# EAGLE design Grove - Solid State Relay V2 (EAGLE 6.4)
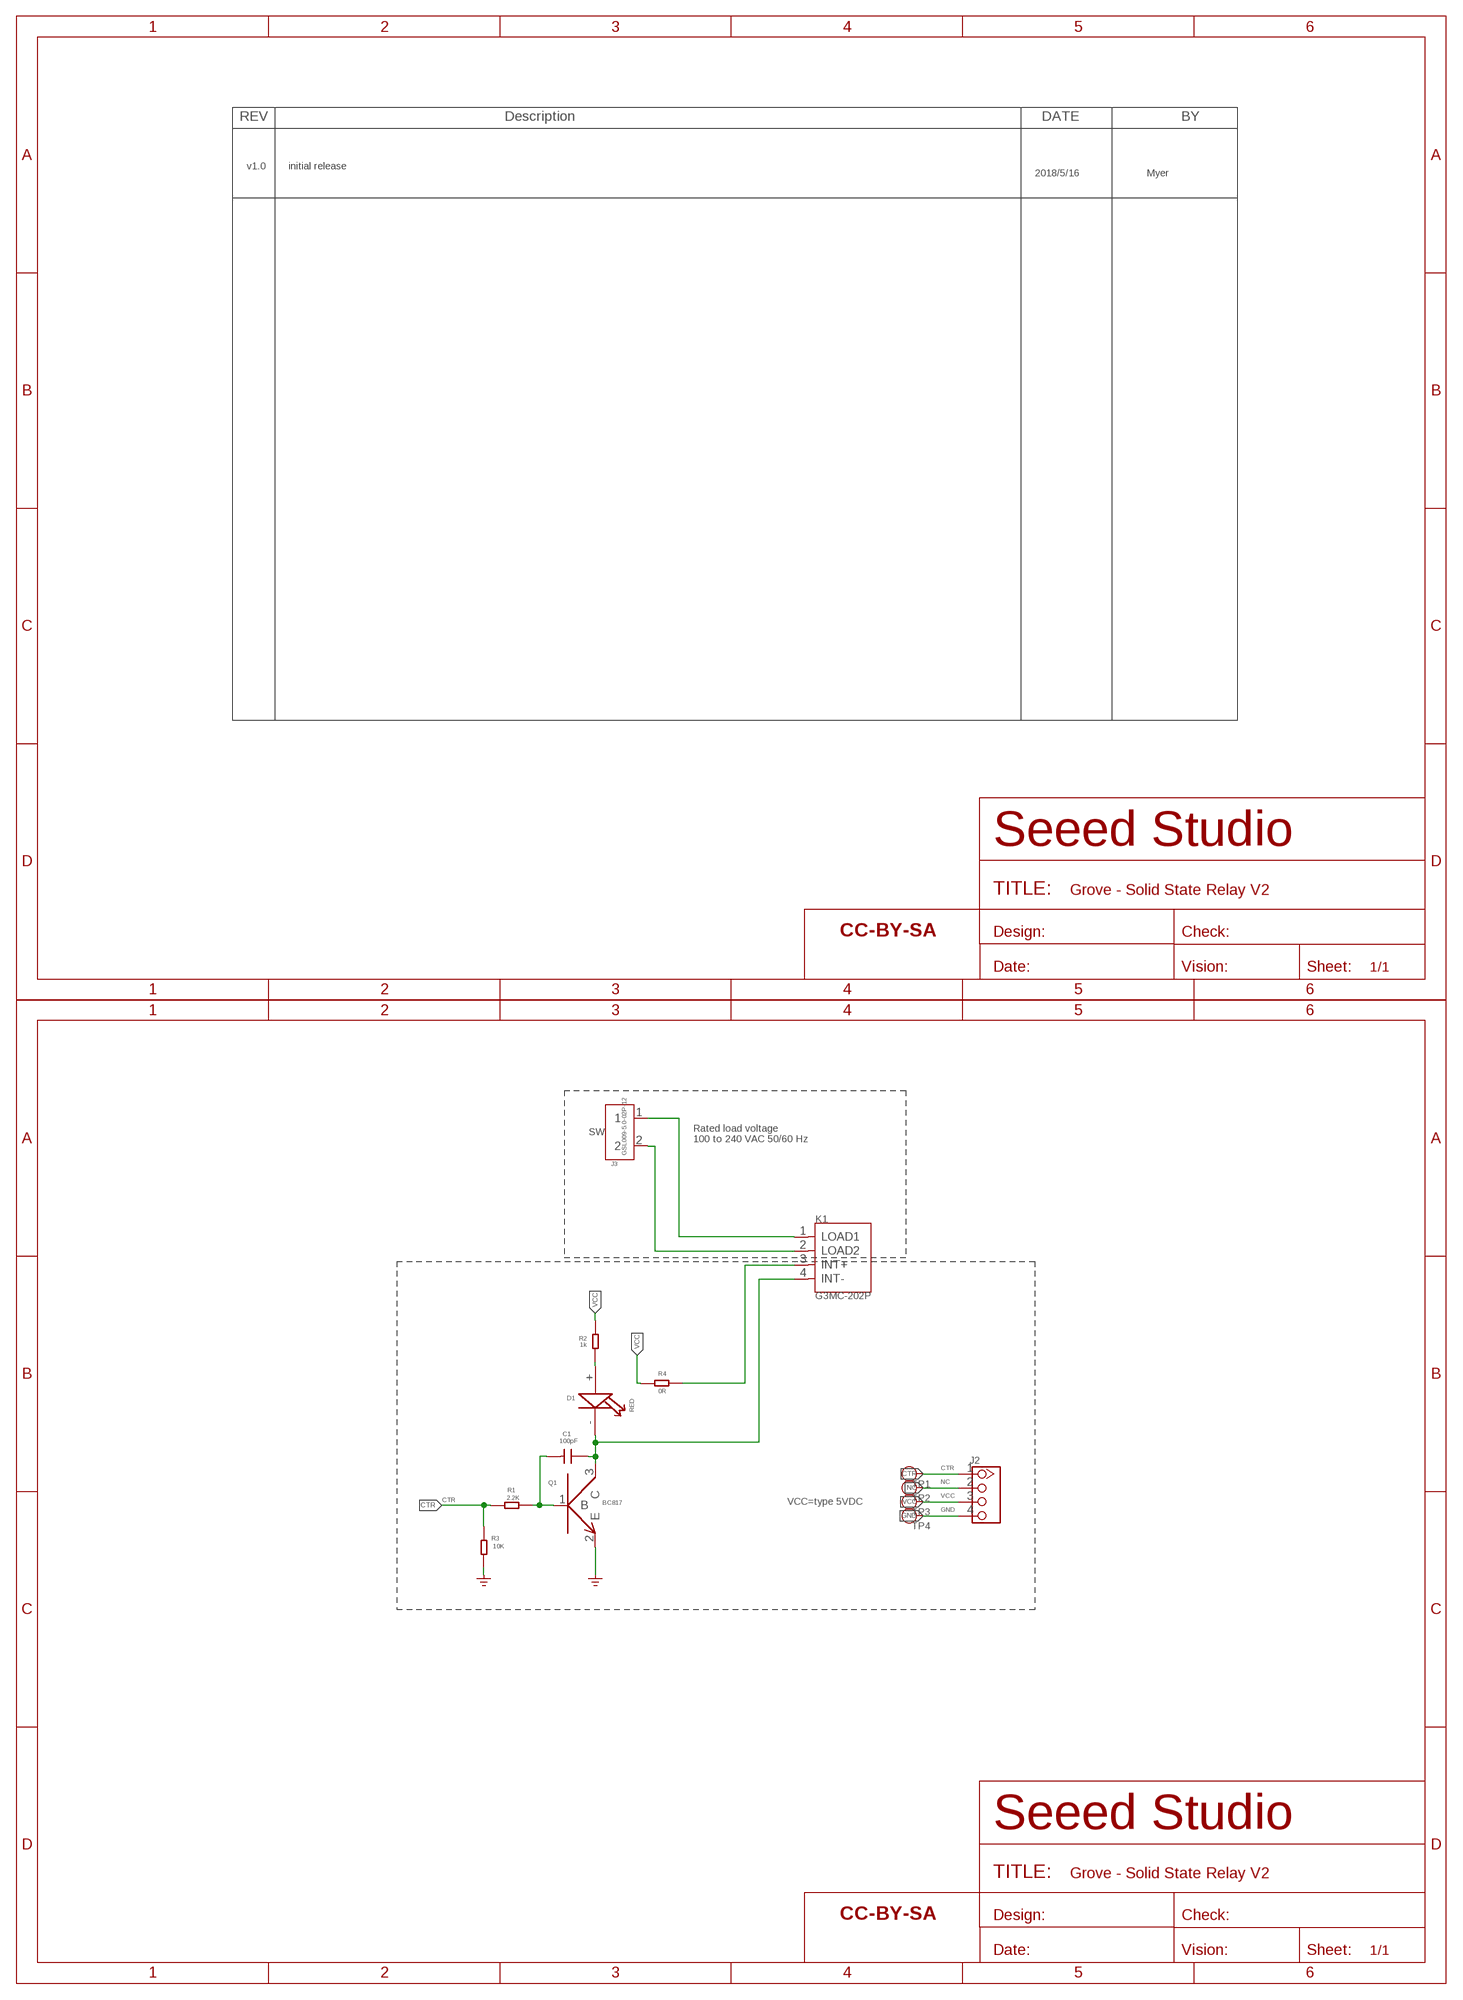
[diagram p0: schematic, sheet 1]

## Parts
C1  100pF  C-0603  [0603]
D1  RED  LED0805  [LED0805]
FR1  SEEEDSTUDIO-OPEN-SCH-FRAME  [SEEEDSTUDIO-PCB-FRAME]
FR2  SEEEDSTUDIO-OPEN-SCH-FRAME  [SEEEDSTUDIO-PCB-FRAME]
J2  TWIG-4P-2.0-2.0  [4P-2.0]
J3  GSL009-5.0-02P-12  SCREW-TERMINAL-2P'5.0-10.6X10X14.8H'  [2P-5.0-10.6X10X14.8H]
K1  G3MC-202P  RELAY-G3MC-201P  [REY4-2.54-24.5X4.5X13.5MM]
Q1  NPN_9013  [SOT23]
R1  2.2K  R-0603  [0603]
R2  1k  R-0603  [0603]
R3  10K  R-0603  [0603]
R4  0R  R-0603  [0603]
TP1  TEST-POINT'4545'  [TP-D45MIL]
TP2  TEST-POINT'4545'  [TP-D45MIL]
TP3  TEST-POINT'4545'  [TP-D45MIL]
TP4  TEST-POINT'4545'  [TP-D45MIL]

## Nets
CTR: J2.1 R1.1 R3.2 TP1.T
GND: J2.4 Q1.2(E) R3.1 TP4.T
N$1: K1.3(INT+) R4.2
N$2: C1.2 Q1.1(B) R1.2
N$3: C1.1 D1.- K1.4(INT-) Q1.3(C)
N$4: J3.2 K1.2(LOAD2)
N$5: J3.1 K1.1(LOAD1)
N$6: D1.+ R2.1
NC: J2.2 TP2.T
VCC: J2.3 R2.2 R4.1 TP3.T

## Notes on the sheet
- v1.0 | initial release
- 2018/5/16 | Myer
- SW
- Rated load voltage 
  100 to 240 VAC 50/60 Hz
- BC817 | VCC=type 5VDC

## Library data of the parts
C1 = Discrete:C*: Ceramic Capacitors
D1 = CPT_SMD:LED0805
FR1 FR2 = moudle-new:SEEEDSTUDIO-OPEN-SCH-FRAME
J2 = Connector:TWIG-4P-2.0
J3 = Connector:SCREW-TERMINAL-2P
K1 = Discrete-new:RELAY-G3MC-201P
Q1 = CPT_SMD:NPN_9013
R1-R4 = Discrete:R*
TP1-TP4 = Discrete-new:TEST-POINT; PARTNO: DNP

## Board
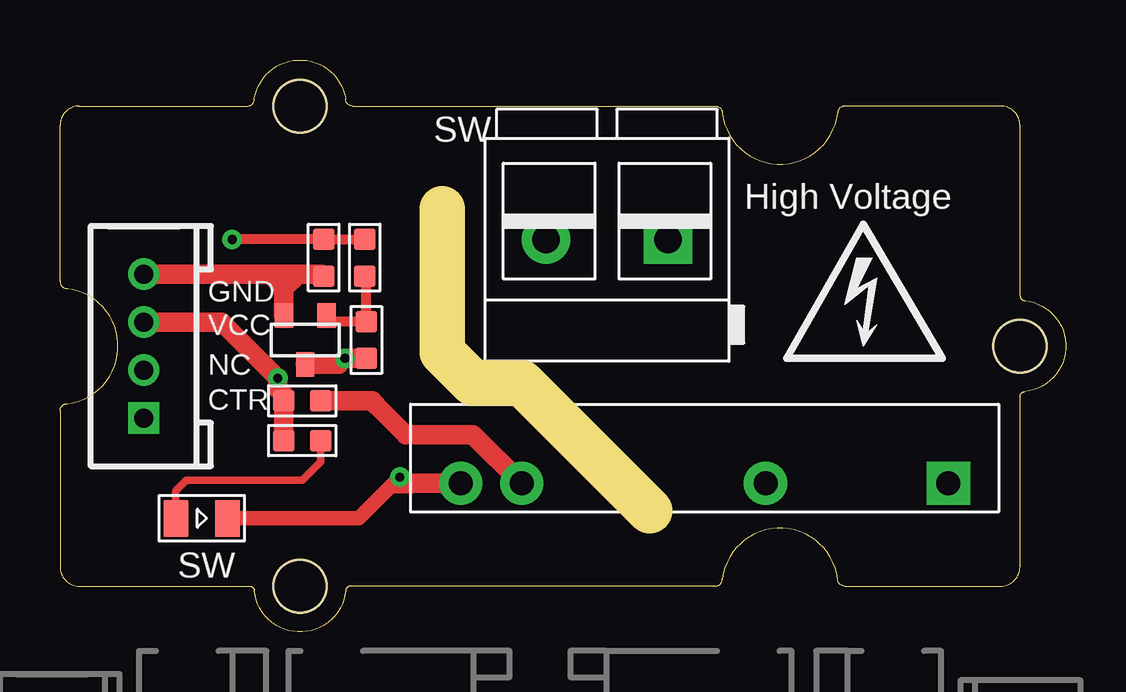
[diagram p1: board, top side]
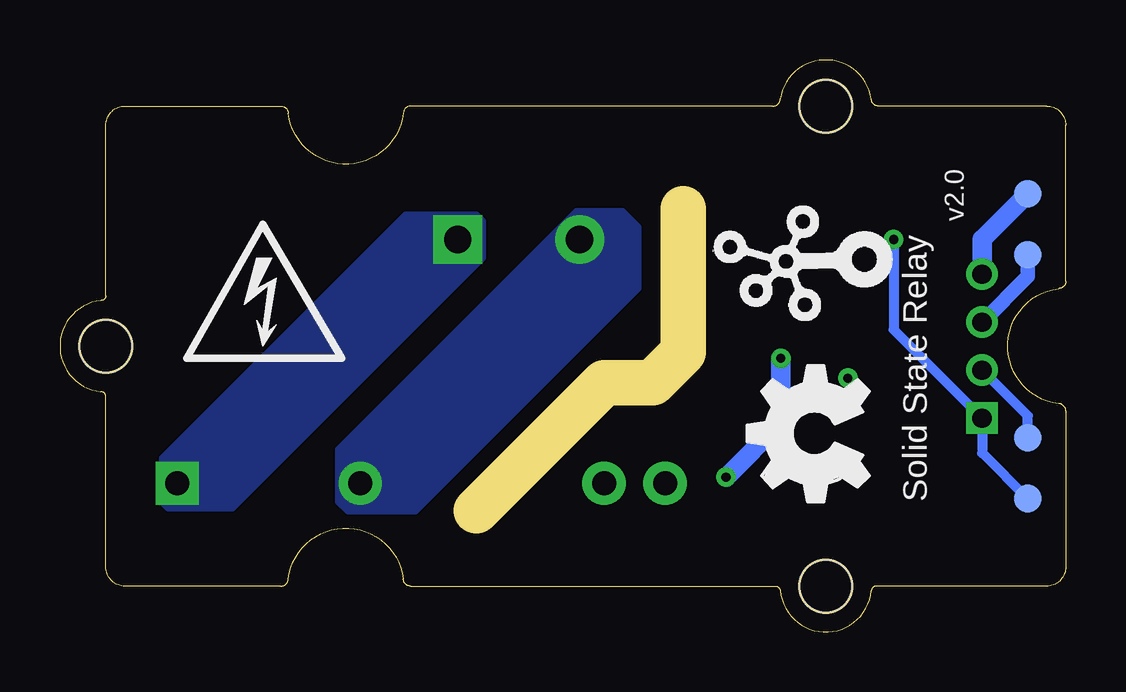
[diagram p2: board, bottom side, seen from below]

Size 41.91 x 23.83 mm. Coordinates in mm from the lower left corner, seen from the top.
Outline: 24.57,5.05 19.24,10.38 17.21,10.38 15.94,11.65 15.94,17.62
Copper layers (1*16): Top 0.035mm / dielectric 1.5mm / Bottom 0.035mm
Design rules "default *": minimum track width 10mil, minimum drill 12mil, track to track 8mil, track to pad 8mil, pad to pad 8mil, via to via 8mil, smd to smd 8mil, copper to edge 10mil, drill to drill 8mil, minimum pad ring 10mil, minimum via ring 8mil, stop-mask expansion 4mil, vias tented up to drill 100mil, thermal gap 10mil

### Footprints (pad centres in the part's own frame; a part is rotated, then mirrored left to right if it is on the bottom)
0603 = smd 0.889 x 0.889: 1 -0.762,0; 2 0.762,0
LED0805 = smd 1.016 x 1.524: + -1.077,0; - 1.077,0
4P-2.0 = drill 0.8 pad 1.27 square: 1 -3,0 | drill 0.8 pad 1.27: 2 -1,0; 3 1,0; 4 3,0
2P-5.0-10.6X10X14.8H = drill 1.143 pad 2.032 square: 1 -2.54,-0.508 | drill 1.143 pad 2.032: 2 2.54,-0.508
REY4-2.54-24.5X4.5X13.5MM = drill 1 pad 1.8 square: 1 -10.16,0 | drill 1 pad 1.8: 2 -2.54,0; 3 7.62,0; 4 10.16,0
SOT23 = smd 0.762 x 1.016: 1 -0.889,-1.016; 2 0.889,-1.016; 3 0,1.016
TP-D45MIL = smd 1.143 x 1.143: T 0,0
GROVE-1*2-TEST-PLATFORM-TOP = hole 2.2: 10.635,10; 10.635,-10; -19.365,0

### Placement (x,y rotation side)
C1  12.76,12.16 90 top
D1  5.9,4.73 0 top
FR1  not placed on the board
FR2  not placed on the board
J2  3.49,11.91 90 top
J3  22.79,15.85 180 top
K1  26.86,6.19 180 top
Q1  10.22,12.16 180 top
R1  12.7,15.59 270 top
R2  10.09,7.97 180 top
R3  10.98,15.59 90 top
R4  10.09,9.62 0 top
TP1  1.59,5.56 180 bottom
TP2  1.59,8.1 180 bottom
TP3  1.59,15.72 180 bottom
TP4  1.59,18.26 180 bottom
U$1  [TWIGLOGO]  8.19,15.46 90 bottom
U$2  [OSHW_FILLX200_NOTEXT]  8.19,5.43 90 bottom
U$6  [GROVE-1*2-TEST-PLATFORM-TOP]  20.64,11.91 180 top

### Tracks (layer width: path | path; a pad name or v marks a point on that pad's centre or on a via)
CTR  (via drill 0.38 pad 0.81)
  Top 0.406: R1.1 R3.2 v7.17,16.35
  Bottom 0.406: TP1.T 3.49,7.46 J2.1 7.17,12.59 v7.17,16.35
GND
  Top 0.813: J2.4 8.75,14.91 | 8.75,14.91 9.33,14.91 | 9.33,14.91 9.92,14.91 | 9.92,14.91 10.9,14.91 R3.1 | Q1.2 9.33,14.32 | 9.33,14.32 9.33,14.91 | 8.75,14.91 9.33,14.32 | 9.92,14.91 9.33,14.32
  Bottom 0.813: J2.4 3.49,16.35 TP4.T
N$1
  Top 0.813: K1.3 17.21,8.23 14.41,8.23 13.21,9.43 13.14,9.5 13.02,9.62 R4.2
N$2
  Top 0.406: R1.2 12.76,14.77 C1.2 11.36,12.92 Q1.1
N$3  (via drill 0.38 pad 0.81)
  Top 0.61: D1.- 12.44,4.73 13.78,6.07 | 13.78,6.07 v14.16,6.45 | 13.78,6.07 14.67,6.07 14.79,6.19
  Top 0.813: C1.1 v11.87,11.4 11.62,11.15 Q1.3 | K1.4 14.79,6.19 14.41,6.19 v14.16,6.45
  Bottom 0.813: v11.87,11.4 11.87,8.73 v14.16,6.45
N$4
  pour Bottom (isolate 0.254, no thermals): 20.38,17.5 18.48,17.5 17.84,16.86 17.84,14.32 27.11,5.05 29.91,5.05 30.29,5.43 30.29,7.59
N$5
  pour Bottom (isolate 0.254, no thermals): 24.32,17.12 24.32,15.59 34.73,5.18 37.4,5.18 37.78,5.56 37.78,7.08 27.49,17.37 24.57,17.37
N$6
  Top 0.305: D1.+ 4.83,5.88 5.27,6.32 10.09,6.32 10.86,7.08 R2.1
NC
  Bottom 0.406: TP2.T 1.59,9 J2.2
VCC  (via drill 0.38 pad 0.81)
  Top 0.813: R2.2 R4.1 9.33,9.88 9.08,10.13 v9.08,10.58 6.75,12.91 J2.3
  Bottom 0.61: TP3.T 1.59,14.81 J2.3

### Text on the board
tPlace: SW | High Voltage | GND | VCC | NC | CTR | SW
bPlace: v2.0 | Solid State Relay

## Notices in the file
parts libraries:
moudle-new: This work is licensed under the Creative Commons Attribution 4.0 International License.
To view a copy of this license,visit:
http://creativecommons.org/licenses/by-sa/4.0
moudle-new: CC-BY-SA
